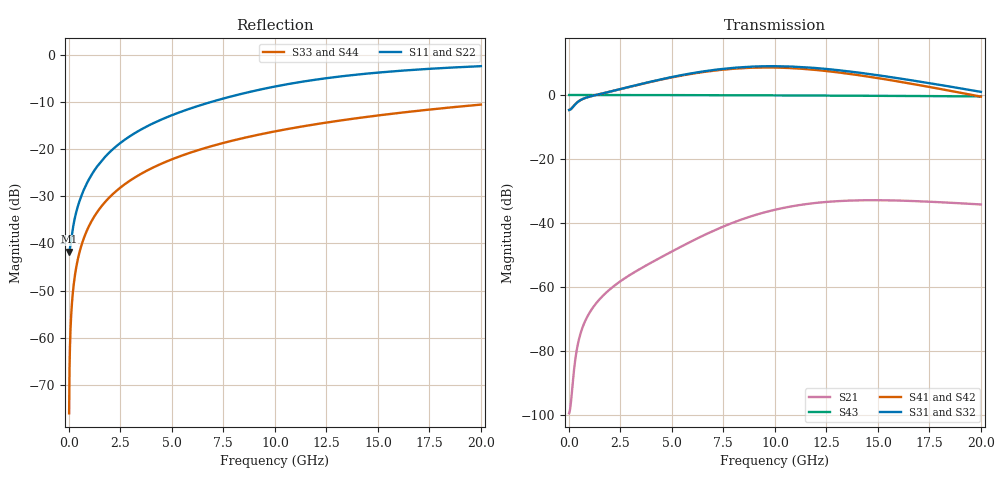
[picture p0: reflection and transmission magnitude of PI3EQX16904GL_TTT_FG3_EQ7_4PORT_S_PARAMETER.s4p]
! NPort=4 DATA=2000 NOISE=0 GROUPDELAY=0 COMPLEX_DATAFORMAT=POLAR
! NumOfBlock=1 NumOfParam=0
! .MODEL Smodel S TSTONEFILE=PI3EQX16904GL_TTT_FG3_EQ7_4PORT_S_PARAMETER.s4p TYPE=S
!  -- The above .MODEL line can be used for the S element in the netlist.
! The s parameter is extracted from the linear redriver, it is not bi-directional; only s(4,1)s(4,2) and s(3,1)s(3,2)
! should be the insertion loss
!Port definition:
!Port1 = input+
!Port2 = input-
!Port3 = output+
!Port4 = output-
# Hz S MA R  50
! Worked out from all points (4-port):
!   2000 points, 10 MHz to 20 GHz, reference 50 ohm
!   strongest paths, dB at 10 MHz, 5.01 GHz, 10.01 GHz, 15.01 GHz, 20 GHz:
!     S31: -4.7, 5.6, 9.0, 6.2, 1.0
!     S32: -4.7, 5.6, 9.0, 6.1, 1.0
!     S41: -4.7, 5.5, 8.6, 5.3, -0.5
!     S42: -4.7, 5.5, 8.6, 5.2, -0.5
!     S43: 0.0, 0.0, -0.1, -0.3, -0.4
!     S21: -99.6, -48.9, -35.9, -32.9, -34.2
!   lowest |S11| = -41.7 dB at 10 MHz (marker M1), VSWR 1.02, Z = 49.2 - j0.0603 ohm
!   |S11| at or under -10 dB: start of sweep to 6.857 GHz
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1e7  0.008182 -175.7  1.05e-05 7.8  0 0.0  0 0.0
     1.05e-05 7.8  0.008182 -175.7  0 0.0  0 0.0
     0.5835 0.7  0.5835 -179.3  0.0001571 -90.0  1 -0.0
     0.5835 -179.3  0.5835 0.7  1 -0.0  0.0001571 -90.0
1e9  0.04923 -106.5  0.0003927 112.3  0 0.0  0 0.0
     0.0003926 112.3  0.04923 -106.5  0 0.0  0 0.0
     0.9434 11.3  0.9441 -168.7  0.01571 -90.9  0.9999 -0.9
     0.943 -170.5  0.9436 9.5  0.9999 -0.9  0.01571 -90.9
5.48e9  0.2524 -103.8  0.004338 110.6  0 0.0  0 0.0
        0.004306 111.0  0.2523 -103.8  0 0.0  0 0.0
        2.051 -30.9  2.036 148.9  0.08574 -95.1  0.996 -4.9
        2.02 139.3  2.006 -40.9  0.996 -4.9  0.08574 -95.1
9.24e9  0.4291 -110.8  0.01393 76.4  0 0.0  0 0.0
        0.01385 77.4  0.4291 -110.8  0 0.0  0 0.0
        2.807 -96.8  2.794 83.2  0.1435 -98.6  0.9888 -8.3
        2.691 67.0  2.679 -113.0  0.9888 -8.3  0.1435 -98.6
1.304e10  0.5895 -120.9  0.02191 25.3  0 0.0  0 0.0
          0.02186 26.7  0.5896 -120.9  0 0.0  0 0.0
          2.452 -167.0  2.444 13.0  0.2003 -102.0  0.9781 -11.6
          2.263 -9.2  2.255 170.7  0.9781 -11.6  0.2003 -102.0
1.619e10  0.6851 -128.8  0.02228 -9.4  0 0.0  0 0.0
          0.02225 -7.8  0.6853 -128.8  0 0.0  0 0.0
          1.787 143.1  1.781 -37.0  0.2459 -104.8  0.9668 -14.2
          1.587 -63.7  1.581 116.1  0.9668 -14.2  0.2459 -104.8
2e10  0.7641 -136.5  0.01942 -38.8  0 0.0  0 0.0
      0.01941 -36.8  0.7644 -136.5  0 0.0  0 0.0
      1.12 92.4  1.116 -87.8  0.2986 -108.1  0.9506 -17.4
      0.943 -119.5  0.9394 60.3  0.9506 -17.4  0.2986 -108.1
